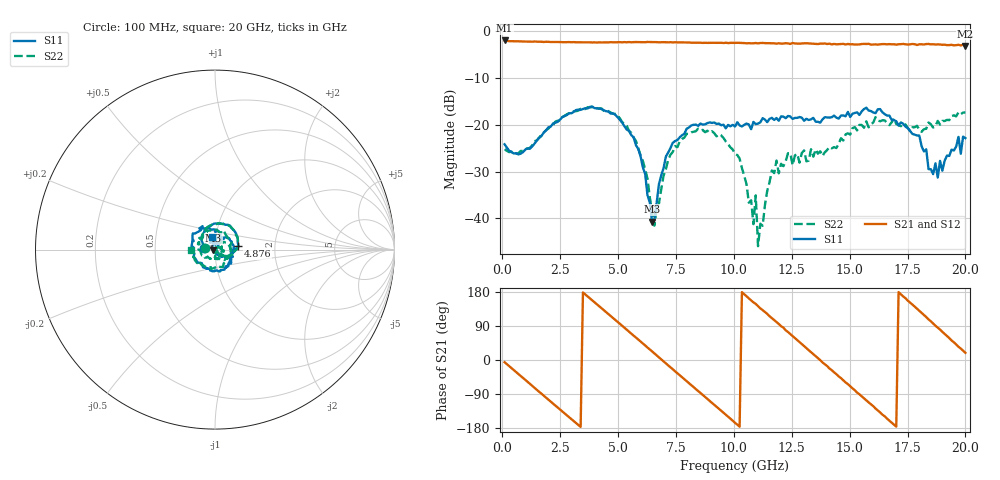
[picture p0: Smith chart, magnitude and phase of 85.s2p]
!Agilent Technologies,N5230C,MY49001569,A.09.33.09
!Agilent N5230C: A.09.33.09
!Date: Monday, July 27, 2015 14:13:52
!Correction: S11(Full 2 Port(1,2))
!S21(Full 2 Port(1,2))
!S12(Full 2 Port(1,2))
!S22(Full 2 Port(1,2))
!S2P File: Measurements: S11, S21, S12, S22:
# Hz S  dB  R 50
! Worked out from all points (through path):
!   201 points, 100 MHz to 20 GHz, reference 50 ohm
!   highest |S21| = -1.92 dB at 100 MHz (marker M1); lowest = -3.1 dB at 20 GHz (marker M2)
!   group delay of S21, straight-line fit = 147 ps
!   lowest |S11| = -40.7 dB at 6.468 GHz (marker M3), VSWR 1.02, Z = 49.2 - j0.361 ohm
!   |S11| at or under -10 dB: start of sweep to end of sweep
!   |S22| runs from -45.9 to -16.2 dB; largest |S21 - S12| = 0.026
!   S11 on the Smith chart (normalised r, x): 100 MHz: 0.88, +0.02; 4.876 GHz: 1.29, +0.06; 20 GHz: 0.96, +0.14
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1e8  -24.14 171.6  -1.92 -5.9  -1.99 -5.7  -25.20 171.9
1.7915e9  -21.60 149.1  -2.24 -94.3  -2.23 -94.1  -21.62 151.4
3.483e9  -16.60 76.4  -2.32 178.3  -2.34 178.1  -16.53 78.8
4.876e9  -17.81 9.4  -2.32 106.2  -2.35 105.8  -17.63 8.8
5.871e9  -25.16 -47.1  -2.28 54.1  -2.27 53.8  -24.90 -36.7
6.468e9  -40.66 -156.6  -2.27 22.8  -2.31 22.4  -38.57 -28.4
6.7665e9  -32.64 133.4  -2.32 6.9  -2.29 6.8  -36.78 62.9
7.264e9  -24.93 84.4  -2.30 -19.5  -2.30 -19.5  -26.37 57.8
8.458e9  -20.19 32.0  -2.39 -81.8  -2.40 -82.3  -20.77 -2.3
1.005e10  -20.33 -17.4  -2.44 -165.7  -2.50 -165.9  -26.19 -76.5
1.0846e10  -19.35 -32.1  -2.52 152.1  -2.46 152.4  -41.23 -86.7
1.09455e10  -19.81 -35.8  -2.47 148.1  -2.48 146.2  -35.06 -77.1
1.1045e10  -19.71 -30.6  -2.55 142.0  -2.45 141.6  -45.93 122.4
1.1841e10  -18.51 -58.1  -2.61 99.9  -2.59 99.2  -27.63 25.3
1.3433e10  -18.48 -124.1  -2.62 15.7  -2.62 15.0  -26.79 -69.1
1.43285e10  -18.00 -161.6  -2.66 -32.4  -2.62 -32.6  -24.74 -121.2
1.51245e10  -17.60 171.5  -2.73 -74.8  -2.72 -75.7  -20.68 179.9
1.67165e10  -18.00 106.2  -2.70 -160.2  -2.69 -160.4  -20.06 75.7
1.801e10  -22.27 50.8  -2.74 129.4  -2.94 129.2  -21.04 -23.7
1.8408e10  -29.45 57.2  -2.67 107.1  -2.80 107.2  -19.48 -65.3
1.9204e10  -26.55 105.6  -2.92 63.5  -2.82 62.9  -18.92 -129.9
2e10  -22.82 102.2  -3.10 19.0  -2.95 17.7  -17.30 179.9
